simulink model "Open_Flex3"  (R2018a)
settings: Solver=VariableStepAuto  StartTime=0.0  StopTime=20.0  RelTol=1e-3
undefined symbols (not defined in the file or in its folder): Af, Ap, Bf, Bp, Cf, Cp, Df, Dp, TVC

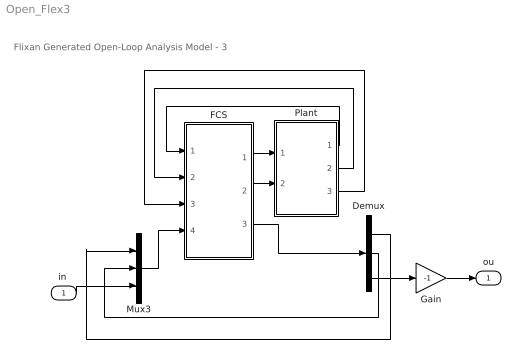
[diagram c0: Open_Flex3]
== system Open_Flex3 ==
  note: Flixan Generated Open-Loop Analysis Model - 3
  "in " : Inport
  Demux : Demux  Outputs=3
  FCS : Subsystem
  Gain : Gain  Gain=-1
  Mux3 : Mux  Inputs=3
  Plant : Subsystem
  ou : Outport
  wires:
  FCS/1(DY) -> Plant/1(Dy)
  FCS/2(DZ) -> Plant/2(Dz)
  Plant/1(attit) -> FCS/1(Attit)
  Plant/2(rate) -> FCS/2(pqr)
  Plant/3(NZY) -> FCS/3(Nzy)
  FCS/3(DQ) -> Demux/1
  Mux3/1 -> FCS/4("DQ ")
  Demux/1 -> Mux3/1
  Gain/1 -> ou/1
  "in "/1 -> Mux3/3
  Demux/3 -> Gain/1
  Demux/2 -> Mux3/2

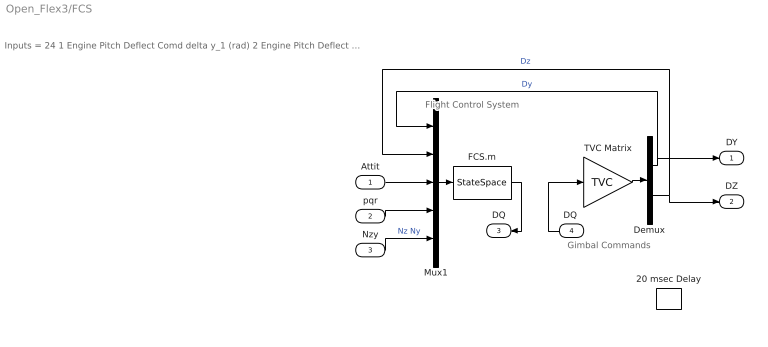
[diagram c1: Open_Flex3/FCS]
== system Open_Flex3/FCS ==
  note: Gimbal Commands
  note: Flight Control System
  note: Inputs = 24 1 Engine Pitch Deflect Comd delta y_1 (rad) 2 Engine Pitch Deflect Comd delta y_2 (rad) 3 Engine Pitch Deflect Comd delta y_3 (rad) 4 Engine Pitch Deflect Comd delta y_4 (rad) 5 Engine Pitch Deflect Comd delta y_5 (rad) 6 Engine Pitch Deflect Comd delta y_6 (rad) 7 Engine Pitch Deflect Comd delta y_7 (rad) 8 Engine Pitch Deflect Comd delta y_8 (rad) 9 Engine Yaw Deflect Commnd delta z_1 (rad) 10 Engine Yaw Deflect Commnd delta z_2 (rad) 11 Engine Yaw Deflect Commnd delta z_3 (rad) 12 Engine Yaw Deflect Commnd delta z_4 (rad) 13 Engine Yaw Deflect Commnd delta z_5 (rad) 14 Engine Yaw Deflect Commnd delta z_6 (rad) 15 Engine Yaw Deflect Commnd delta z_7 (rad) 16 Engine Yaw Deflect Commnd delta z_8 (rad) 17 Roll Attitude Error (rad) 18 Pitch Attitude Error (rad) 19 Yaw Attitude Error (rad) 20 Roll Rate (rad/sec) 21 Pitch Rate (rad/sec) 22 Yaw Rate (rad/sec) 23 Normal Acceleration NZ (ft/sec^2) 24 Lateral Acceleration NY (ft/sec^2)
  Attit : Inport
  pqr : Inport  Port=2
  Nzy : Inport  Port=3
  "DQ " : Inport  Port=4
  20 msec Delay : TransportDelay  DelayTime="[1  1  1]*0.02"  InitialOutput="[0  0  0]"  PadeOrder=2
  Demux : Demux  Outputs=[8, 8]
  FCS.m : StateSpace  A=Af  B=Bf  C=Cf  D=Df  InitialCondition=0
  Mux1 : Mux  Inputs=[8, 8, 3, 3, 2]
  TVC Matrix : Gain  Gain=TVC  Multiplication=Matrix(K*u)
  DY : Outport
  DZ : Outport  Port=2
  DQ : Outport  Port=3
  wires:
  Demux/1 -> Mux1/1, DY/1  "Dy"
  Demux/2 -> DZ/1, Mux1/2  "Dz"
  Nzy/1 -> Mux1/5  "Nz Ny"
  Attit/1 -> Mux1/3
  pqr/1 -> Mux1/4
  Mux1/1 -> FCS.m/1
  TVC Matrix/1 -> Demux/1
  "DQ "/1 -> TVC Matrix/1
  FCS.m/1 -> DQ/1

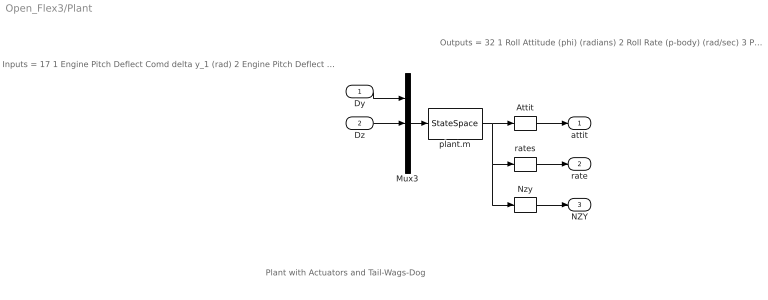
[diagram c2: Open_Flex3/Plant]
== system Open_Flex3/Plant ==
  note: Inputs = 17 1 Engine Pitch Deflect Comd delta y_1 (rad) 2 Engine Pitch Deflect Comd delta y_2 (rad) 3 Engine Pitch Deflect Comd delta y_3 (rad) 4 Engine Pitch Deflect Comd delta y_4 (rad) 5 Engine Pitch Deflect Comd delta y_5 (rad) 6 Engine Pitch Deflect Comd delta y_6 (rad) 7 Engine Pitch Deflect Comd delta y_7 (rad) 8 Engine Pitch Deflect Comd delta y_8 (rad) 9 Engine Yaw Deflect Commnd delta z_1 (rad) 10 Engine Yaw Deflect Commnd delta z_2 (rad) 11 Engine Yaw Deflect Commnd delta z_3 (rad) 12 Engine Yaw Deflect Commnd delta z_4 (rad) 13 Engine Yaw Deflect Commnd delta z_5 (rad) 14 Engine Yaw Deflect Commnd delta z_6 (rad) 15 Engine Yaw Deflect Commnd delta z_7 (rad) 16 Engine Yaw Deflect Commnd delta z_8 (rad) 17 Wind-Gust Velocity (ft/sec)
  note: Outputs = 32 1 Roll Attitude (phi) (radians) 2 Roll Rate (p-body) (rad/sec) 3 Pitch Attitude (thet) (radians) 4 Pitch Rate (q-body) (rad/sec) 5 Yaw Attitude (psi) (radians) 6 Yaw Rate (r-body) (rad/sec) 7 Angle of attack, alfa, (radian) 8 Angle of sideslip, beta, (radian) 9 Change in Altitude, delta-h, (feet) 10 Forward Acceleration (V-dot) (ft/sec) 11 Cross Range Velocity (Vcr) (ft/sec) 12 Rate-Gyro # 1, Roll Rate (Body) (rad/sec) 13 Rate-Gyro # 2, Pitch Rate (Body) (rad/sec) 14 Rate-Gyro # 3, Yaw Rate (Body) (rad/sec) 15 Accelerom # 1, (along Y), (ft/sec^2) Translat. Accelerat. 16 Accelerom # 2, (along Z), (ft/sec^2) Translat. Accelerat. 17 Engine #1 Pitch Deflection dy-1 (rad) 18 Engine #2 Pitch Deflection dy-2 (rad) 19 Engine #3 Pitch Deflection dy-3 (rad) 20 Engine #4 Pitch Deflection dy-4 (rad) 21 Engine #5 Pitch Deflection dy-5 (rad) 22 Engine #6 Pitch Deflection dy-6 (rad) 23 Engine #7 Pitch Deflection dy-7 (rad) 24 Engine #8 Pitch Deflection dy-8 (rad) 25 Engine #1 Yaw Deflection dz-1 (rad) 26 Engine #2 Yaw Deflection dz-2 (rad) 27 Engine #3 Yaw Deflection dz-3 (rad) 28 Engine #4 Yaw Deflection dz-4 (rad) 29 Engine #5 Yaw Deflection dz-5 (rad) 30 Engine #6 Yaw Deflection dz-6 (rad) 31 Engine #7 Yaw Deflection dz-7 (rad) 32 Engine #8 Yaw Deflection dz-8 (rad)
  note: Plant with Actuators and Tail-Wags-Dog
  Dy : Inport
  Dz : Inport  Port=2
  Attit : Selector  InputPortWidth=32  IndexOptions=Index vector (dialog)  Indices=[1,3,5]  OutputSizes=1
  Mux3 : Mux  Inputs=[8, 8, 1]
  Nzy : Selector  InputPortWidth=32  IndexOptions=Index vector (dialog)  Indices=[16,15]  OutputSizes=1
  plant.m : StateSpace  A=Ap  B=Bp  C=Cp  D=Dp  InitialCondition=0
  rates : Selector  InputPortWidth=32  IndexOptions=Index vector (dialog)  Indices=[12,13,14]  OutputSizes=1
  attit : Outport
  rate : Outport  Port=2
  NZY : Outport  Port=3
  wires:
  Nzy/1 -> NZY/1
  Attit/1 -> attit/1
  Mux3/1 -> plant.m/1
  plant.m/1 -> Nzy/1, rates/1, Attit/1
  rates/1 -> rate/1
  Dz/1 -> Mux3/2
  Dy/1 -> Mux3/1
